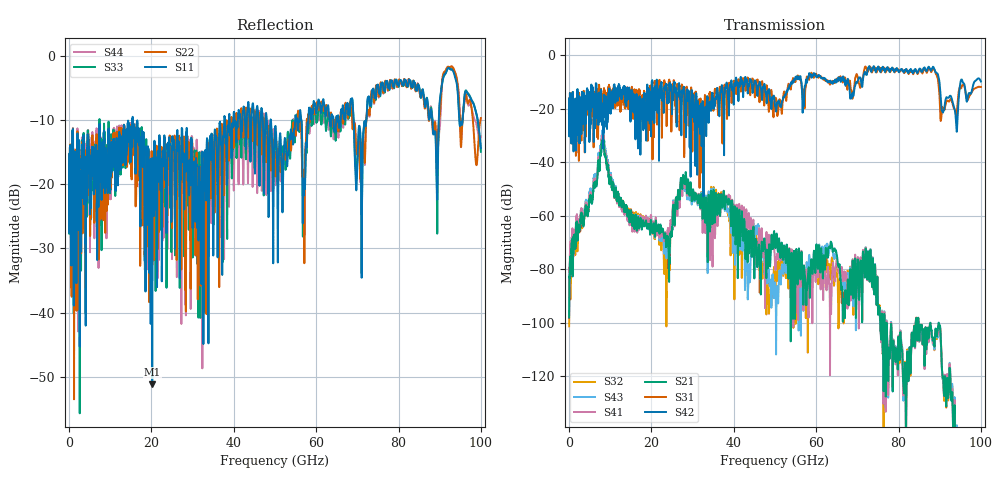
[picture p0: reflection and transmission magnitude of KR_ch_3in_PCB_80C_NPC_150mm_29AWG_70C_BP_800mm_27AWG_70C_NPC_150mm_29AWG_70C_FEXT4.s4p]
# GHz S RI R 45
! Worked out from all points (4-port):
!   4000 points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, 25 MHz to 100 GHz, reference 45 ohm
!   strongest paths, dB at 25 MHz, 25.02 GHz, 50.02 GHz, 75.03 GHz, 100 GHz:
!     S42: -21.8, -20.6, -18.8, -4.2, -9.7
!     S31: -21.7, -12.4, -15.9, -5.0, -11.8
!     S21: -98.1, -65.0, -71.4, -95.7, -174.9
!     S41: -90.3, -61.1, -78.9, -95.7, -179.4
!     S43: -97.2, -61.2, -85.3, -95.5, -180.8
!     S32: -101.4, -62.1, -85.2, -95.4, -173.4
!   lowest |S11| = -51.2 dB at 20.2 GHz (marker M1), VSWR 1.01, Z = 45.1 - j0.215 ohm
!   |S11| at or under -10 dB: start of sweep to 15.35 GHz; 15.48 GHz to 37.69 GHz (22.21 GHz wide, 83.6 % of centre); 48.99 GHz to 54.9 GHz (5.906 GHz wide, 11.4 % of centre)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
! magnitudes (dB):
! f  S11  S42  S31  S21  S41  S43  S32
! 25 MHz  -17.2  -21.8  -21.7  -98.1  -90.3  -97.2  -101.4
! 8.1 GHz  -13.5  -18.8  -19.0  -32.0  -30.3  -28.3  -29.9
! 20.2 GHz  -51.2  -9.2  -14.2  -66.0  -66.5  -65.9  -65.6
! 23.5 GHz  -17.6  -11.9  -13.9  -69.4  -68.3  -71.0  -78.9
! 28.05 GHz  -19.8  -15.9  -19.4  -48.1  -49.4  -50.6  -49.5
! 46.73 GHz  -8.1  -13.6  -10.4  -71.3  -65.0  -68.1  -77.0
! 100 GHz  -14.3  -9.7  -11.8  -174.9  -179.4  -180.8  -173.4
